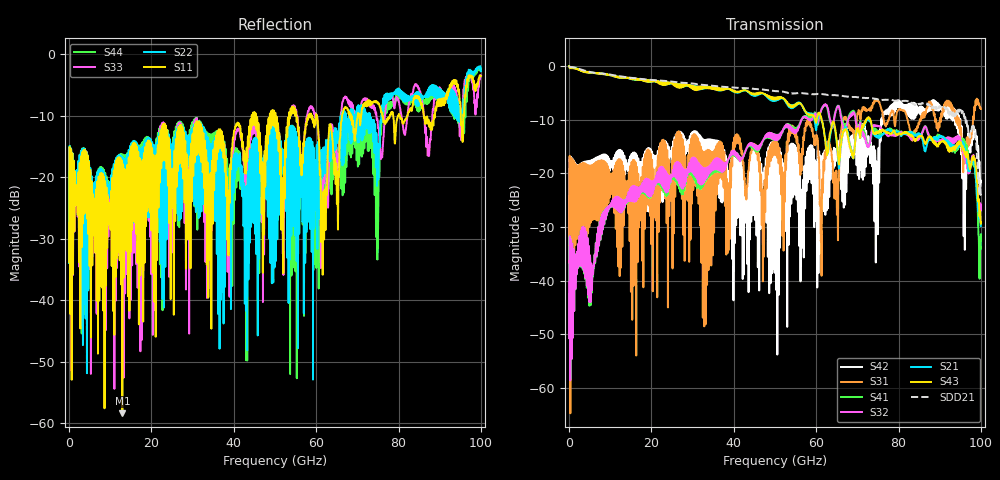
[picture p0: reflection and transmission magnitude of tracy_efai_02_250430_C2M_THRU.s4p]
!! PART DESCRIPTION: TE 224G+ VSR Channel- Chip to module, IO connector to CPC(Co-packaged connector) through over the board cable
!! CHANNEL DESCRIPTION: Module trace -> Mated IO 224G+ Connector -> Internal Cable Termination -> 30AWG 300mm Cable -> Cable
!!  termination + CPC connector(No footprint or package included)
!! MODEL REVISION:  Rev 3, Created on April 25, 2025
!! MODEL STATUS: Development
!! MODEL GEOMETRY: 8 Pair Channel
!! MODEL FREQUENCY RANGE: 0 GHz to 100 GHz in 10.00 MHz frequency steps
!! MODEL EDGE RATE LIMITATION: 5ps (Using conservative 0.5/Fmax rule of thumb)
!! PORT DEFINITIONS:
!! Port  1  ----->  Module Side  -->  Host Side, A Row  <-----  Port  2
!! Port  3  ----->  Module Side  -->  Host Side, A Row  <-----  Port  4
# GHz S MA R 45
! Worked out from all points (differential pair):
!   10000 points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, 10 MHz to 100 GHz, reference 45 ohm
!   strongest paths, dB at 10 MHz, 25.01 GHz, 50.01 GHz, 75.01 GHz, 100 GHz:
!     S43: -0.1, -3.3, -6.2, -12.4, -29.2
!     S21: -0.1, -3.3, -6.5, -13.1, -29.8
!     S32: -50.7, -20.7, -12.8, -11.2, -25.8
!     S41: -50.7, -21.1, -12.9, -12.5, -31.4
!     S31: -36.5, -18.1, -14.5, -6.3, -8.0
!     S42: -36.7, -15.5, -15.5, -28.4, -21.6
!   taken as a pair (ports 3,1 in; 4,2 out), SDD21 dB: 0.0, -2.9, -4.7, -6.3, -23.3
!   lowest |S11| = -58.4 dB at 12.94 GHz (marker M1), VSWR 1.00, Z = 44.9 - j0.0695 ohm
!   |S11| at or under -10 dB: start of sweep to 44.34 GHz; 45.38 GHz to 48.72 GHz (3.339 GHz wide, 7.1 % of centre); 60.11 GHz to 66.29 GHz (6.181 GHz wide, 9.78 % of centre)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
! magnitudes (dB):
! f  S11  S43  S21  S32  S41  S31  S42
! 10 MHz  -33.8  -0.1  -0.1  -50.7  -50.7  -36.5  -36.7
! 12.94 GHz  -58.4  -2.1  -2.1  -26.2  -26.3  -32.7  -21.8
! 51.98 GHz  -30.4  -6.0  -6.1  -11.8  -11.9  -21.7  -21.7
! 54.3 GHz  -9.5  -7.4  -7.4  -11.9  -11.5  -12.5  -23.0
! 62.14 GHz  -22.8  -13.3  -13.2  -7.3  -7.3  -16.1  -17.9
! 95.78 GHz  -9.7  -15.6  -14.9  -16.3  -13.9  -18.7  -22.9
! 100 GHz  -3.5  -29.2  -29.8  -25.8  -31.4  -8.0  -21.6
